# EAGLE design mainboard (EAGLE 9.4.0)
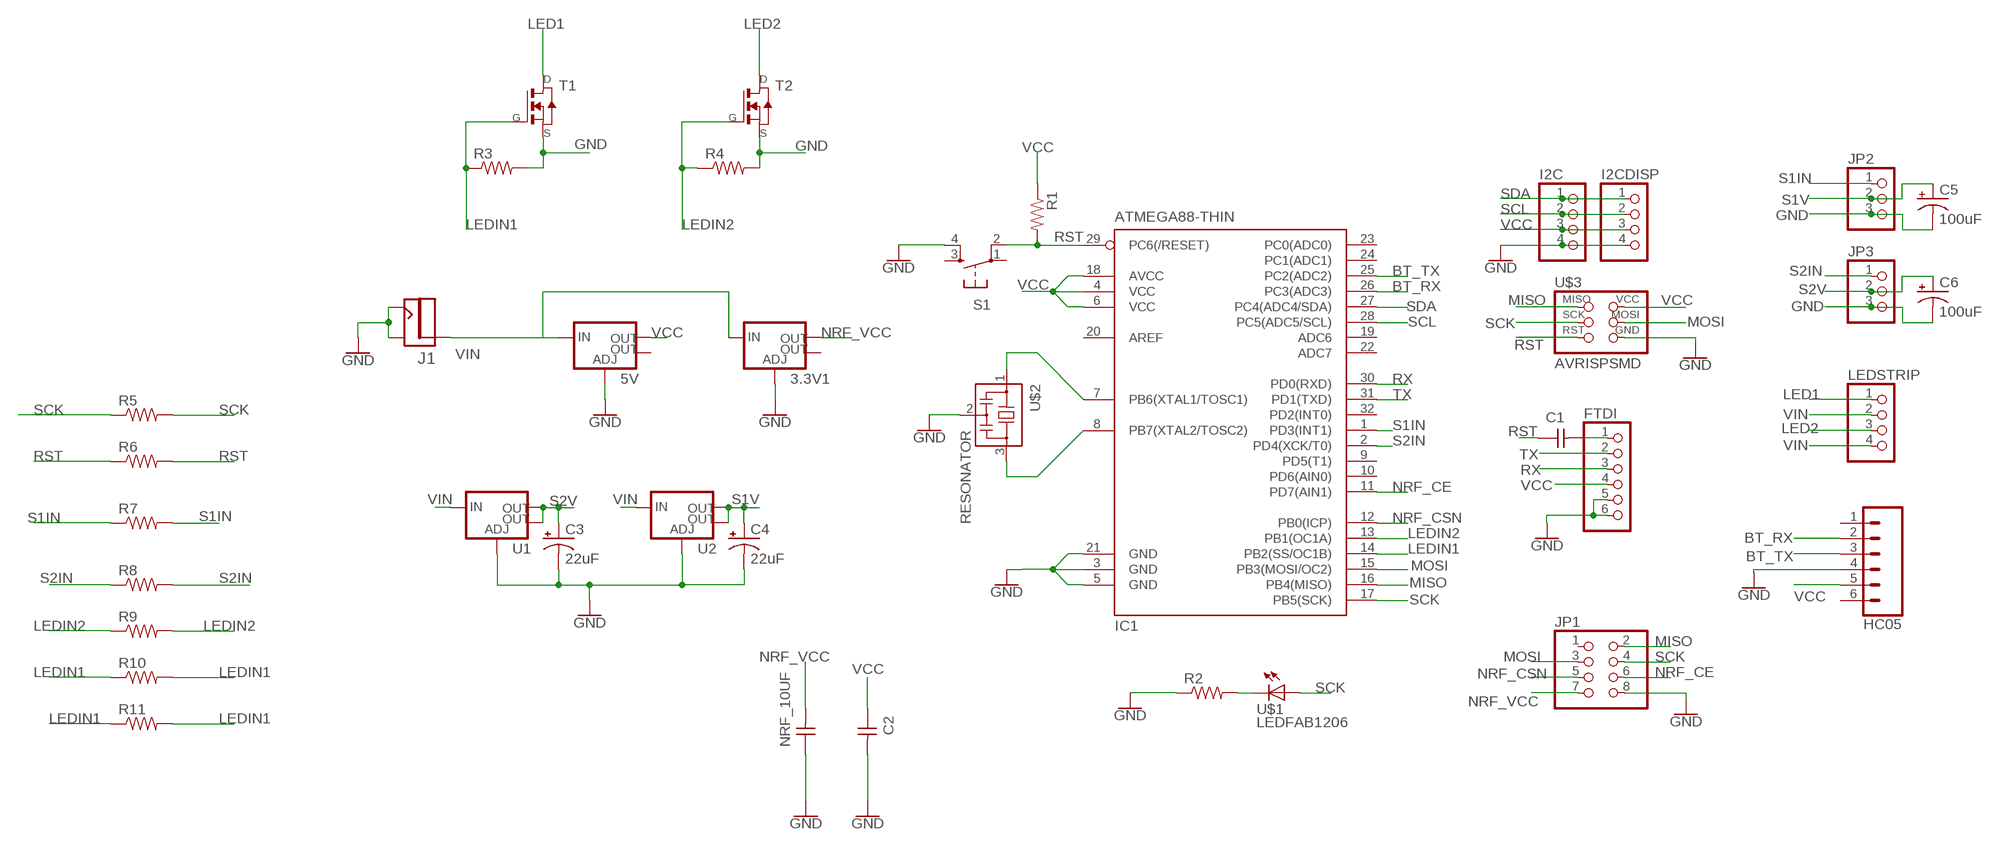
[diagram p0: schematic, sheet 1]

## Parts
3.3V1  V_REG_LM1117SOT223  [SOT223]
5V  V_REG_LM1117SOT223  [SOT223]
C1  CAP-UNPOLARIZEDFAB  [C1206FAB]
C2  CAP-UNPOLARIZEDFAB  [C1206FAB]
C3  22uF  22UF-POLAR-PANASONIC_C-35V-20%  [PANASONIC_C]
C4  22uF  22UF-POLAR-PANASONIC_C-35V-20%  [PANASONIC_C]
C5  100uF  100UF-POLAR-25V-20%(ELEC)  [PANASONIC_D]
C6  100uF  100UF-POLAR-25V-20%(ELEC)  [PANASONIC_D]
FTDI  PINHD-1X61X06_SMT  [1X06_SMT]
HC05  CONN_06SMD-FEMALE-V2  [1X06-SMD-FEMALE]
I2C  PINHD-1X41X04_SMT  [1X04_SMT]
I2CDISP  PINHD-1X41X04_SMT  [1X04_SMT]
IC1  ATMEGA88-THIN  [TQFP32-08THIN]
J1  JACK2.1MM  [JACK_2.1MM]
JP1  PINHD-2X4SMT  [2X04_SMT]
JP2  PINHD-1X31X03_SMT  [1X03_SMT]
JP3  PINHD-1X31X03_SMT  [1X03_SMT]
LEDSTRIP  PINHD-1X41X04_SMT  [1X04_SMT]
NRF_10UF  CAP-UNPOLARIZEDFAB  [C1206FAB]
R1  RES-US1206FAB  [R1206FAB]
R2  RES-US1206FAB  [R1206FAB]
R3  RES-US1206FAB  [R1206FAB]
R4  RES-US1206FAB  [R1206FAB]
R5  RES-US1206FAB  [R1206FAB]
R6  RES-US1206FAB  [R1206FAB]
R7  RES-US1206FAB  [R1206FAB]
R8  RES-US1206FAB  [R1206FAB]
R9  RES-US1206FAB  [R1206FAB]
R10  RES-US1206FAB  [R1206FAB]
R11  RES-US1206FAB  [R1206FAB]
S1  6MM_SWITCH6MM_SWITCH  [6MM_SWITCH]
T1  NMOSFETSOT23  [SOT-23]
T2  NMOSFETSOT23  [SOT-23]
U1  V_REG_LM1117SOT223  [SOT223]
U2  V_REG_LM1117SOT223  [SOT223]
U$1  LEDFAB1206  [LED1206FAB]
U$2  RESONATOR  [EFOBM]
U$3  AVRISPSMD  [2X03SMD]

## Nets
BT_RX: HC05.2 IC1.26(PC3(ADC3))
BT_TX: HC05.3 IC1.25(PC2(ADC2))
GND: 3.3V1.1(ADJ) 5V.1(ADJ) C2.2 C3.- C4.- C5.- C6.- FTDI.5 FTDI.6 HC05.4 I2C.4 I2CDISP.4 IC1.3(GND) IC1.5(GND) IC1.21(GND) J1.CONTACT J1.SHUNT JP1.8 JP2.3 JP3.3 NRF_10UF.1 R2.1 R3.2 R4.2 S1.4(S1) T1.2(S) T2.2(S) U1.1(ADJ) U2.1(ADJ) U$2.2 U$3.6(GND)
LED1: LEDSTRIP.1 T1.1(D)
LED2: LEDSTRIP.3 T2.1(D)
LEDIN1: IC1.14(PB2(SS/OC1B)) R3.1 R10.1 R10.2 R11.1 R11.2 T1.3(G)
LEDIN2: IC1.13(PB1(OC1A)) R4.1 R9.1 R9.2 T2.3(G)
MISO: IC1.16(PB4(MISO)) JP1.2 U$3.1(MISO)
MOSI: IC1.15(PB3(MOSI/OC2)) JP1.3 U$3.4(MOSI)
N$1: IC1.7(PB6(XTAL1/TOSC1)) U$2.1
N$2: IC1.8(PB7(XTAL2/TOSC2)) U$2.3
N$5: C1.2 FTDI.1
N$18: R2.2 U$1.2(C)
NRF_CE: IC1.11(PD7(AIN1)) JP1.6
NRF_CSN: IC1.12(PB0(ICP)) JP1.5
NRF_VCC: 3.3V1.2(OUT) JP1.7 NRF_10UF.2
RST: C1.1 IC1.29(PC6(/RESET)) R1.2 R6.1 R6.2 S1.2(P1) U$3.5(RST)
RX: FTDI.3 IC1.30(PD0(RXD))
S1IN: IC1.1(PD3(INT1)) JP2.1 R7.1 R7.2
S1V: C4.+ C5.+ JP2.2 U2.2(OUT) U2.4(OUT)
S2IN: IC1.2(PD4(XCK/T0)) JP3.1 R8.1 R8.2
S2V: C3.+ C6.+ JP3.2 U1.2(OUT) U1.4(OUT)
SCK: IC1.17(PB5(SCK)) JP1.4 R5.1 R5.2 U$1.1(A) U$3.3(SCK)
SCL: I2C.2 I2CDISP.2 IC1.28(PC5(ADC5/SCL))
SDA: I2C.1 I2CDISP.1 IC1.27(PC4(ADC4/SDA))
TX: FTDI.2 IC1.31(PD1(TXD))
VCC: 5V.2(OUT) C2.1 FTDI.4 HC05.5 I2C.3 I2CDISP.3 IC1.4(VCC) IC1.6(VCC) IC1.18(AVCC) R1.1 U$3.2(VCC)
VIN: 3.3V1.3(IN) 5V.3(IN) J1.PIN LEDSTRIP.2 LEDSTRIP.4 U1.3(IN) U2.3(IN)
Unconnected: 3.3V1.4(OUT) 5V.4(OUT) HC05.1 HC05.6 IC1.9(PD5(T1)) IC1.10(PD6(AIN0)) IC1.19(ADC6) IC1.20(AREF) IC1.22(ADC7) IC1.23(PC0(ADC0)) IC1.24(PC1(ADC1)) IC1.32(PD2(INT0)) JP1.1 S1.1(P) S1.3(S)

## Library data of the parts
3.3V1 5V U1 U2 = fab:V_REG_LM1117: Voltage Regulator LM1117 Standard adjustable voltage regulator but in SMD form. Spark Fun Electronics SKU : COM-00595; PROD_ID: VREG-08170
C1 C2 NRF_10UF = fab:CAP-UNPOLARIZED
C3 C4 = SparkFun-Capacitors:22UF-POLAR: 22µF polarized capacitors; PROD_ID: CAP-08618
C5 C6 = SparkFun-Capacitors:100UF-POLAR: 100µF polarized capacitors; PROD_ID: CAP-12547
FTDI = smd_con:PINHD-1X6: PIN HEADER
HC05 = SparkFun-Connectors:CONN_06: Multi connection point. Often used as Generic Header-pin footprint for 0.1 inch spaced/style header connections On any of the 0.1 inch spaced packages, you can populate with these: Break Away Headers - Straight (PRT-00116) Break Away Male Headers - Right Angle (PRT-00553) Female Headers (PRT-00115)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; PROD_ID: CONN-09668
I2C I2CDISP LEDSTRIP = smd_con:PINHD-1X4: PIN HEADER
IC1 = fab:ATMEGA88-THIN
J1 = fab:JACK
JP1 = smd_con:PINHD-2X4: PIN HEADER
JP2 JP3 = smd_con:PINHD-1X3: PIN HEADER
R1-R11 = fab:RES-US: Resistor (US Symbol)
S1 = fab:6MM_SWITCH: OMRON SWITCH
T1 T2 = fab:NMOSFET: MOS FET
U$1 = fab:LED: LED
U$2 = fab:RESONATOR
U$3 = fab:AVRISP

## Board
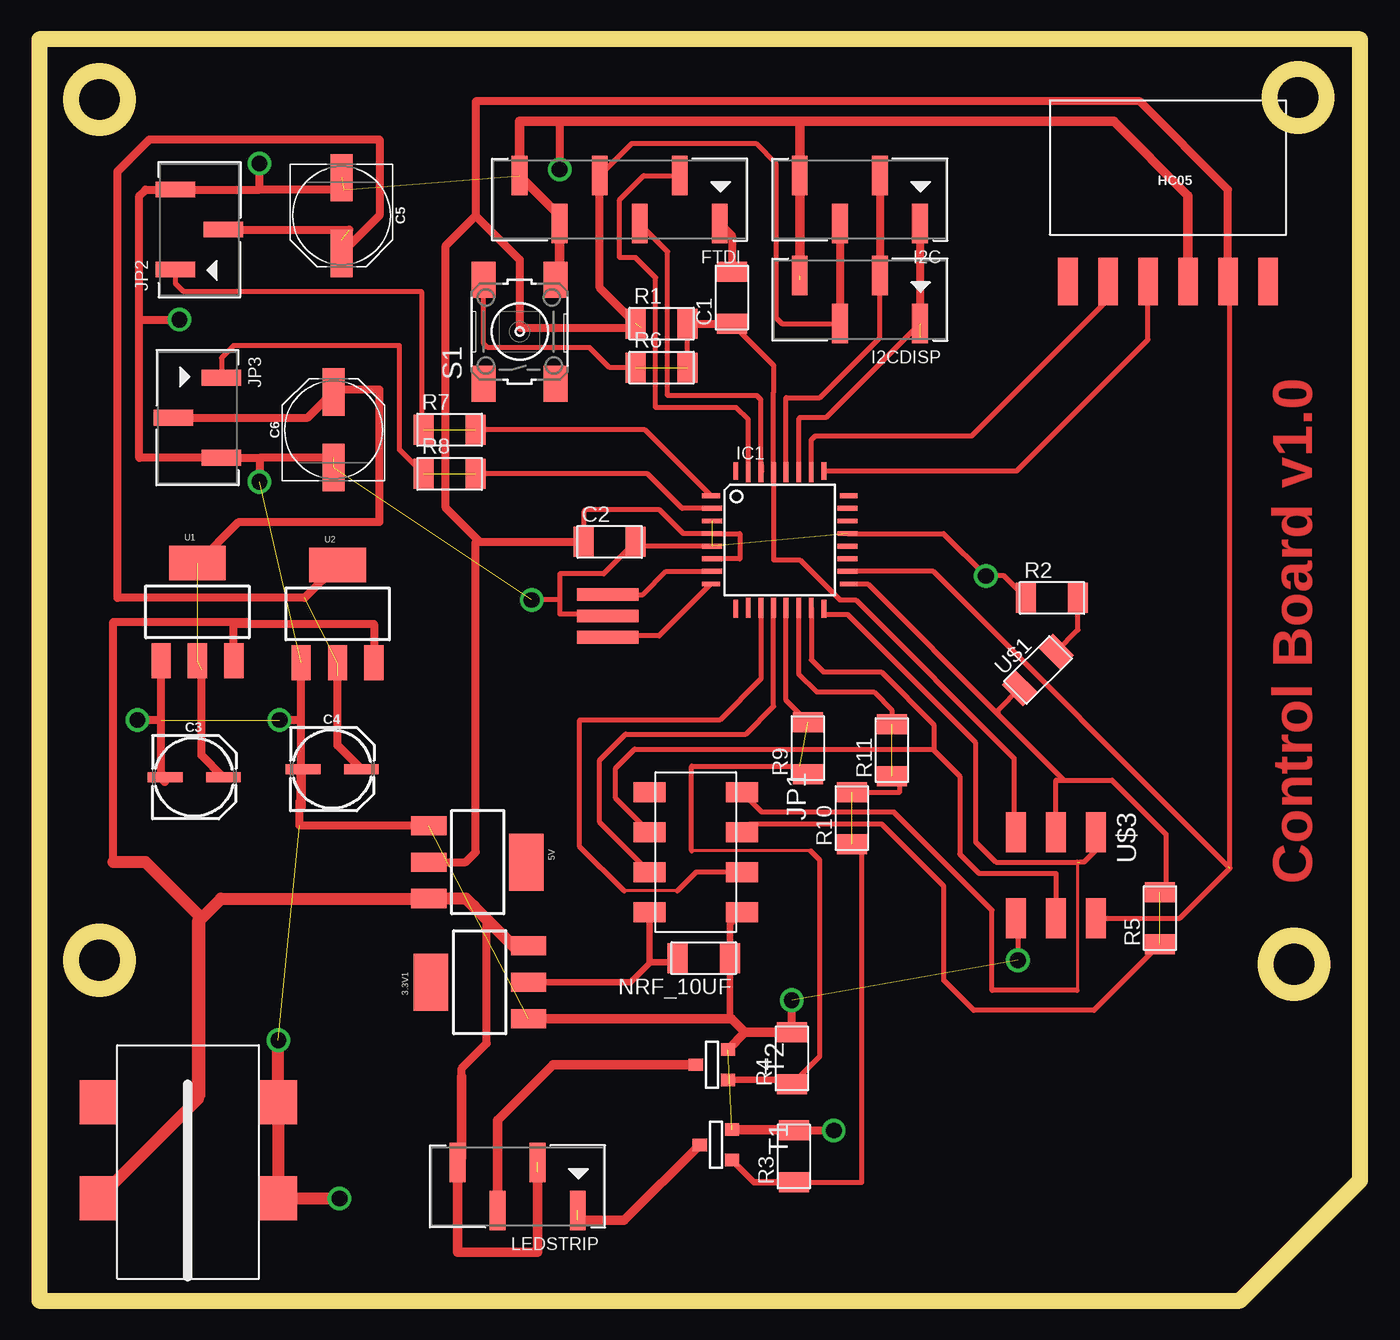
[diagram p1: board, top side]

Size 83.82 x 80.01 mm. Coordinates in mm from the lower left corner, seen from the top.
Outline: 0,0 76.2,0 83.82,7.62 83.82,80.01 0,80.01 0,0
Outline: circle at 79.63,21.34 radius 1.8
Outline: circle at 3.81,21.59 radius 1.8
Outline: circle at 3.81,76.2 radius 1.8
Outline: circle at 79.88,76.33 radius 1.8
Copper layers (1*16): Top 0.035mm / dielectric 1.5mm / Bottom 0.035mm
Design rules "default *": minimum track width 6mil, minimum drill 0.35mm, track to track 16mil, track to pad 16mil, pad to pad 16mil, via to via 16mil, smd to smd 16mil, copper to edge 40mil, drill to drill 6mil, minimum pad ring 10mil, minimum via ring 8mil, stop-mask expansion 4mil, vias tented up to drill 0mil, thermal gap 10mil

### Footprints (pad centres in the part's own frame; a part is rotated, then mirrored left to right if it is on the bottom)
SOT223 = smd 1.219 x 2.235: 1 -2.311,-3.099; 2 0,-3.099; 3 2.311,-3.099 | smd 3.6 x 2.2: 4 0,3.099
C1206FAB = smd 1.27 x 1.905: 1 -1.651,0; 2 1.651,0
PANASONIC_C = smd 2.2 x 0.65: + 1.9,-0.2; - -1.8,-0.2
PANASONIC_D = smd 3 x 1.4: + 2.4,0; - -2.4,0
1X06_SMT = smd 1 x 2.5: 1 -6.35,1.52; 2 -3.81,-1.52; 3 -1.27,1.52; 4 1.27,-1.52; 5 3.81,1.52; 6 6.35,-1.52
1X06-SMD-FEMALE = smd 1.25 x 3: 1 6.35,3.425; 2 3.81,3.425; 3 1.27,3.425; 4 -1.27,3.425; 5 -3.81,3.425; 6 -6.35,3.425
1X04_SMT = smd 1 x 2.5: 1 -3.81,1.52; 2 -1.27,-1.52; 3 1.27,1.52; 4 3.81,-1.52
TQFP32-08THIN = smd 1.118 x 0.305: 1 -4.369,2.8; 8 -4.369,-2.8; 17 4.369,-2.8; 24 4.369,2.8 | smd 1.27 x 0.305: 2 -4.293,2; 3 -4.293,1.2; 4 -4.293,0.4; 5 -4.293,-0.4; 6 -4.293,-1.2; 7 -4.293,-2; 18 4.293,-2; 19 4.293,-1.2; 20 4.293,-0.4; 21 4.293,0.4; 22 4.293,1.2; 23 4.293,2 | smd 0.305 x 1.118: 9 -2.8,-4.369; 16 2.8,-4.369; 25 2.8,4.369; 32 -2.8,4.369 | smd 0.305 x 1.27: 10 -2,-4.293; 11 -1.2,-4.293; 12 -0.4,-4.293; 13 0.4,-4.293; 14 1.2,-4.293; 15 2,-4.293; 26 2,4.293; 27 1.2,4.293; 28 0.4,4.293; 29 -0.4,4.293; 30 -1.2,4.293; 31 -2,4.293
JACK_2.1MM = smd 2.388 x 2.794: CONTACT 5.766,-2.413; PIN -5.639,-2.413; PIN1 -5.639,3.683; SHUNT 5.766,3.683
2X04_SMT = smd 1.27 x 2.032: 1 -3.81,-2.921; 2 -3.81,2.921; 3 -1.27,-2.921; 4 -1.27,2.921; 5 1.27,-2.921; 6 1.27,2.921; 7 3.81,-2.921; 8 3.81,2.921
1X03_SMT = smd 1 x 2.5: 1 -2.54,1.52; 2 0,-1.52; 3 2.54,1.52
R1206FAB = smd 1.27 x 1.905: 1 -1.651,0; 2 1.651,0
6MM_SWITCH = smd 2.286 x 1.524: 1 -3.302,2.286; 2 3.302,2.286; 3 -3.302,-2.286; 4 3.302,-2.286
SOT-23 = smd 0.787 x 0.889: 1 0.025,-1.016; 2 -0.94,1.016; 3 0.991,1.016
LED1206FAB = smd 1.27 x 1.905: 1 -1.651,0; 2 1.651,0
EFOBM = smd 0.8 x 3.9: 1 -1.35,0; 2 0,0; 3 1.35,0
2X03SMD = smd 2.54 x 1.27: 1 -2.54,2.54; 2 2.92,2.54; 3 -2.54,0; 4 2.92,0; 5 -2.54,-2.54; 6 2.92,-2.54

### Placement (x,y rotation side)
3.3V1  27.94,20.19 90 top
5V  27.81,27.81 270 top
C1  43.94,63.63 90 top
C2  36.2,48.13 0 top
C3  9.78,33.4 0 top
C4  18.54,33.91 0 top
C5  19.18,68.83 270 top
C6  18.67,55.25 90 top
FTDI  36.83,69.85 180 top
HC05  71.63,68.07 180 top
I2C  52.07,69.85 180 top
I2CDISP  52.07,63.5 180 top
IC1  46.99,48.26 0 top
J1  9.4,8.89 0 top
JP1  41.66,28.45 270 top
JP2  10.16,67.94 90 top
JP3  10.03,56.01 270 top
LEDSTRIP  30.35,7.24 180 top
NRF_10UF  42.16,21.72 180 top
R1  39.5,61.98 0 top
R2  64.26,44.58 0 top
R3  47.88,9.14 90 top
R4  47.75,15.37 90 top
R5  71.12,24.26 90 top
R6  39.5,59.18 0 top
R7  26.04,55.25 0 top
R8  26.04,52.45 0 top
R9  48.77,35.05 90 top
R10  51.56,30.61 90 top
R11  54.1,34.92 90 top
S1  30.48,61.47 90 top
T1  42.93,9.91 270 top
T2  42.67,14.99 270 top
U1  10.03,43.69 0 top
U2  18.92,43.56 0 top
U$1  63.37,40 45 top
U$2  36.07,43.43 270 top
U$3  64.52,27.18 270 top

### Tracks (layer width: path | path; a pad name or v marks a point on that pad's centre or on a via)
BT_RX
  Top 0.305: IC1.26 48.99,54.61 49.24,54.86 59.18,54.86 67.82,63.5 HC05.2
BT_TX
  Top 0.305: IC1.25 62.03,52.63 70.36,60.96 HC05.3
GND  (via drill 1)  (13 unrouted)
  Top 0.305: IC1.5 38.12,47.86 C2.2 35.81,46.1 33.02,46.1 33.02,44.45 | 33.02,44.45 33.02,43.56 35.94,43.56 U$2.2 | 33.02,44.45 v31.24,44.45 | R2.1 61.21,45.97 v60.07,45.97 57.39,48.66 IC1.21 | U$3.6 62.1,24.13 v62.1,21.59
  Top 0.406: JP1.8 43.82,23.88 NRF_10UF.1 43.82,18.14 43.56,17.88
  Top 0.508: 7.72,36.83 7.72,33.46 C3.- 7.98,32.89 7.85,33.02 | 7.72,36.83 U1.1 | C4.- 16.61,33.84 16.61,36.83 | 16.61,36.83 U2.1 | 13.97,70.48 JP2.3 6.73,70.48 6.35,70.1 6.35,62.23 | 19.3,70.48 13.97,70.48 | 13.97,53.47 JP3.3 6.35,53.47 6.35,62.23 | 18.67,53.47 13.97,53.47 | 6.35,62.23 v8.89,62.23 | 16.61,36.83 v15.24,36.83 | 7.72,36.83 v6.22,36.83 | 33.02,74.8 v33.02,71.75 | 5V.1 16.51,30.12 16.51,31.65 16.61,31.75 | 13.97,53.47 v13.97,51.94 | 13.97,70.48 v13.97,72.14 | R4.2 v47.75,19.05 | R3.2 v50.42,10.79
  Top 0.61: S1.4 33.02,65.02 FTDI.5 33.02,68.83 FTDI.6 30.48,74.8 33.02,74.8 48.26,74.8 | 48.26,74.8 I2C.4 48.26,64.77 | 48.26,74.8 68.2,74.8 72.9,70.1 HC05.4 | 16.61,31.29 16.61,31.75 16.61,33.84 | T2.2 44.78,17.02 | 44.78,17.02 R4.2 | T1.2 47.83,10.85 R3.2 | 3.3V1.1 43.56,17.88 43.92,17.88 44.78,17.02
  Top 0.762: v19.05,6.48 J1.CONTACT J1.SHUNT v15.16,16.51
LED1  (1 unrouted)
  Top 0.61: T1.1 37.11,5.08 34.16,5.08
LED2
  Top 0.61: LEDSTRIP.3 29.08,11.43 32.61,14.96 T2.1
LEDIN1  (2 unrouted)
  Top 0.305: R3.1 52.2,7.49 52.2,28.96 R10.1 | R10.2 54.61,32.26 54.61,32.77 R11.1 | IC1.14 48.19,39.75 49.33,38.61 52.96,38.61 54.1,37.47 R11.2
  Top 0.406: T1.3 45.36,7.49 R3.1
LEDIN2  (1 unrouted)
  Top 0.203: 48.95,28.52 41.4,28.52
  Top 0.305: R4.1 49.53,15.49 49.53,27.94 48.95,28.52 | 41.4,28.52 41.4,33.91 48.26,33.91 R9.1 | R9.2 47.39,38.08 IC1.13
  Top 0.406: T2.3 47.47,14 R4.1
MISO  (1 unrouted)
  Top 0.203: 65.86,27.81 65.86,19.69
  Top 0.305: U$3.1 67.06,28.57 66.29,27.81 66.04,27.81 | 65.86,27.81 60.71,27.81 59.44,29.08 59.44,35.39 51.31,43.51 49.79,43.51 IC1.16 | 65.86,19.69 60.45,19.69 60.45,24.77 54.24,30.99 45.85,30.99 JP1.2
MOSI
  Top 0.305: 56.69,34.98 58.42,33.25 58.42,28.32 59.64,27.1 64.52,27.1 U$3.4 | JP1.3 36.58,31.88 36.58,33.78 37.77,34.98 56.69,34.98 | 56.69,34.98 56.77,34.98 56.77,36.54 53.43,39.88 49.75,39.88 48.99,40.64 IC1.15
N$1
  Top 0.305: U$2.1 38.31,44.78 39.78,46.26 IC1.7
N$2
  Top 0.305: IC1.8 39.33,42.16 36.15,42.16 U$2.3
N$5
  Top 0.508: FTDI.1 43.94,67.57 C1.2
N$18
  Top 0.305: U$1.2 65.91,42.55 R2.2
NRF_CE
  Top 0.203: 40.49,25.98 37.11,25.98
  Top 0.305: 37.11,25.98 34.29,28.8 34.29,36.83 43.18,36.83 45.79,39.44 IC1.11 | JP1.6 41.68,27.18 40.49,25.98
NRF_CSN
  Top 0.305: JP1.5 35.56,30.35 35.56,34.29 37.21,35.94 44.83,35.94 46.59,37.7 IC1.12
NRF_VCC
  Top 0.406: 38.79,21.46 38.73,21.46 JP1.7 | 38.79,21.46 37.52,20.19 3.3V1.2 | 38.79,21.46 40.51,21.46 NRF_10UF.2
RST  (1 unrouted)
  Top 0.305: U$3.5 61.85,29.84 61.85,34.42 51.82,44.45 50.8,44.45 48.26,46.99 46.61,46.99 46.59,47.01 IC1.29 46.59,57.64 46.61,57.66 46.61,59.31 C1.1 | R6.2 R1.2 | R6.1 36.2,59.18 34.92,60.45 28.45,60.45 28.19,60.71 S1.2
  Top 0.508: R1.2 C1.1
RX
  Top 0.305: 45.83,52.93 45.83,52.59 IC1.30 45.79,57.15 45.54,57.4 39.88,57.4 39.88,66.55 FTDI.3
S1IN  (1 unrouted)
  Top 0.305: IC1.1 38.44,55.25 R7.2 | R7.1 24.26,55.37 24.26,64.01 9.14,64.01 8.64,64.51 JP2.1
S1V  (3 unrouted)
  Top 0.508: C4.+ 18.92,35.23 18.92,39.62 | JP2.2 19.68,67.94 | U2.4 16.84,44.58 4.95,44.58 4.95,71.63 6.98,73.66 21.59,73.66 21.59,68.85 C5.+
  Top 0.61: 19.18,66.04 C5.+ 19.18,67.31
S2IN  (1 unrouted)
  Top 0.305: R8.2 38.61,52.45 40.8,50.26 IC1.2 | R8.1 22.86,53.97 22.86,60.58 12.32,60.58 11.55,59.81 JP3.1
S2V  (2 unrouted)
  Top 0.508: C3.+ 10.29,34.59 10.29,40 | JP3.2 17.03,56.01 C6.+ 18.81,57.78 21.59,57.78 21.59,49.4 12.65,49.4 U1.4
SCK  (1 unrouted)
  Top 0.305: IC1.17 52.58,45.46 60.83,37.21 | U$3.3 64.52,33.02 65.02,33.02 | 60.83,37.21 65.02,33.02 | U$1.1 60.83,37.47 60.83,37.21 | 65.02,33.02 68.07,33.02 71.5,29.59 71.5,26.29 R5.2 | R5.1 66.93,18.41 59.31,18.41 57.4,20.32 57.4,26.29 53.47,30.23 45.09,30.23 JP1.4
SCL
  Top 0.305: IC1.28 47.39,57.28 49.53,57.28 53.34,61.09 53.34,64.77
  Top 0.508: I2C.2 I2CDISP.2 53.34,64.77
SDA  (1 unrouted)
  Top 0.305: I2CDISP.1 49.91,56.01 48.26,56.01 48.19,55.94 IC1.27
  Top 0.508: I2C.1 55.88,60.96
TX
  Top 0.305: FTDI.2 38.35,71.37 36.83,69.85 36.83,66.17 37.85,66.17 39.12,64.9 39.12,56.65 44.22,56.65 44.99,55.88 IC1.31
VCC  (2 unrouted)
  Top 0.305: FTDI.4 37.6,73.41 45.47,73.41 46.74,72.14 46.74,62.36 47.11,61.98 I2CDISP.3 | C2.1 34.54,50.04 34.67,50.17 39.37,50.17 40.88,48.66 IC1.4 44.45,48.66 44.45,47.06 IC1.6 | U$3.2 72.39,24.26 75.56,27.43 75.56,64.52 HC05.5 | 75.44,27.56 56.74,46.26 IC1.18
  Top 0.508: 5V.2 27.05,27.81 27.69,28.45 27.69,48.13 27.94,48.13 | 27.94,48.13 C2.1 | I2C.3 I2CDISP.3 | HC05.5 75.44,70.48 69.85,76.07 27.69,76.07 27.69,68.83 | 27.69,68.83 30.48,66.04 30.48,61.72 38.23,61.72 | R1.1 35.56,64.26 FTDI.4 | 27.94,48.13 25.78,50.29 25.78,66.93 27.69,68.83
VIN  (1 unrouted)
  Top 0.508: U1.3 12.34,42.91 12.36,42.91 | 13.34,42.91 21.23,42.91 U2.3 | 13.34,42.91 12.36,42.91 | 12.34,42.93 12.36,42.91 | 26.8,14.22 26.8,14.73 28.38,16.32 28.38,24.19 | 10.07,12.79 10.29,13.01 10.29,24.26 | 5V.3 11.53,25.5 | 4.7,27.81 4.7,43.05 13.19,43.05 13.34,42.91
  Top 0.61: 31.62,8.13 31.62,3.05 26.54,3.05 LEDSTRIP.4 26.8,9.01 26.8,14.22 | 5V.3 25.4,25.5 | 27.56,25.02 28.38,24.19 30.35,22.23
  Top 0.762: J1.PIN 10.07,12.79 10.07,24.04 10.29,24.26 | 10.29,24.26 6.73,27.81 4.7,27.81 | 10.29,24.26 11.53,25.5 25.4,25.5 | 3.3V1.3 30.07,22.5 27.56,25.02 27.08,25.5 25.4,25.5 | 5V.3 25.4,25.5

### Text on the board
Top: Control Board v1.0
